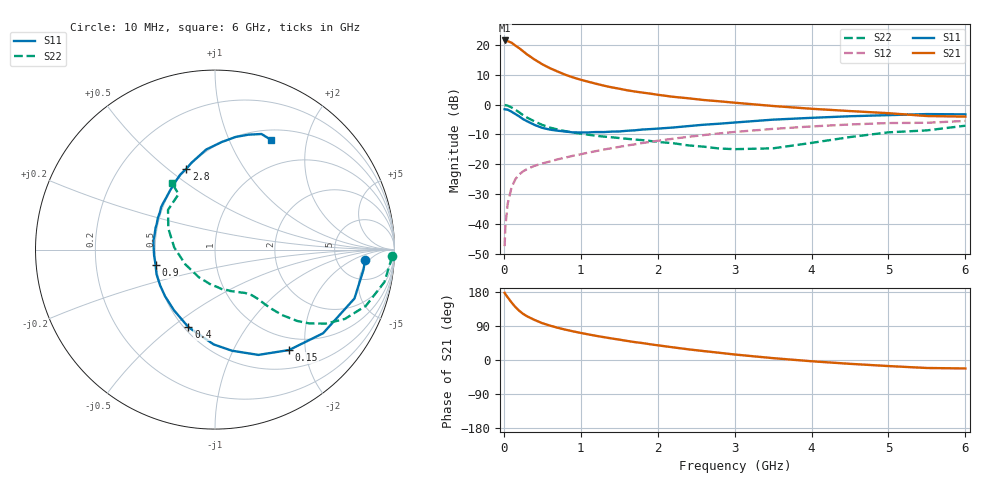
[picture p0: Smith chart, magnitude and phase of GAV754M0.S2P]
! Infineon Technologies  Discrete & RF Semiconductors
! BF775
! Si NPN RF Bipolar Junction Transistor in SOT23
! VCE = 0.75 V  IC = 4 mA
! Common Emitter S-Parameters:  May  1996
# GHz  S  MA  R  50
!  f  S11  S21  S12  S22
! GHz  MAG  ANG  MAG  ANG  MAG  ANG  MAG  ANG
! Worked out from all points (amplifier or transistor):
!   36 points, 10 MHz to 6 GHz, reference 50 ohm
!   highest |S21| = 21.6 dB at 10 MHz (marker M1)
!   |S21| within 3 dB of that: start of sweep to 219.7 MHz
!   unconditionally stable (mu >= 1): 769.2 MHz to end of sweep
!   at 250 MHz: K = 0.46, MSG = 20.2 dB, |S12| = -22.4 dB
!   at 1.4 GHz: K = 1.19, MAG = 7.6 dB, |S12| = -14.6 dB
!   at 6 GHz: K = 1.06, MAG = -0.8 dB, |S12| = -5.5 dB
!   S11 on the Smith chart (normalised r, x): 10 MHz: 10, -4; 150 MHz: 0.78, -1.70; 400 MHz: 0.53, -0.57; 900 MHz: 0.50, -0.09; 2.8 GHz: 0.50, +0.58; 6 GHz: 0.62, +1.44
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0.01  0.8385 -3.9  11.97 177.3  0.0042 87.3  0.9869 -2.2
0.02  0.8347 -7.8  11.78 173.9  0.009 84.9  0.9791 -4.4
0.05  0.8234 -19.3  11.64 165.4  0.0217 80.0  0.9613 -10.8
0.1  0.7617 -37.7  10.98 151.9  0.0407 70.8  0.8975 -20.4
0.15  0.6952 -53.6  9.805 139.7  0.056 62.6  0.8202 -28.1
0.2  0.6346 -67.6  8.869 130.0  0.0673 57.7  0.7429 -33.7
0.25  0.5712 -80.5  7.895 121.8  0.0758 53.7  0.6664 -38.1
0.3  0.5284 -90.8  7 115.5  0.0826 51.4  0.6081 -40.9
0.4  0.4564 -109.0  5.721 105.6  0.094 48.3  0.5221 -44.3
0.5  0.4078 -124.2  4.763 97.2  0.1028 47.4  0.4564 -46.3
0.6  0.3805 -137.1  4.096 90.7  0.1113 47.4  0.4118 -47.6
0.7  0.3651 -146.8  3.589 85.1  0.1206 47.4  0.3826 -48.4
0.9  0.3418 -165.7  2.863 75.6  0.1385 47.6  0.3409 -50.2
1.1  0.3417 178.6  2.419 67.5  0.1567 48.2  0.3119 -52.9
1.3  0.3462 166.5  2.085 60.3  0.176 48.1  0.2909 -55.8
1.6  0.364 151.0  1.744 50.4  0.2057 47.1  0.2671 -61.9
2.2  0.4129 127.5  1.355 33.4  0.2677 42.9  0.2254 -79.4
2.8  0.4784 109.4  1.139 19.1  0.3289 36.7  0.1834 -107.7
3.5  0.5599 95.0  0.949 4.9  0.3916 27.7  0.1847 -153.7
4.5  0.6387 79.5  0.78 -10.1  0.4647 14.6  0.2855 155.6
5.5  0.6942 68.1  0.644 -21.1  0.4962 1.0  0.3697 123.3
6  0.6865 63.2  0.63 -22.3  0.5328 -2.7  0.4428 122.9
